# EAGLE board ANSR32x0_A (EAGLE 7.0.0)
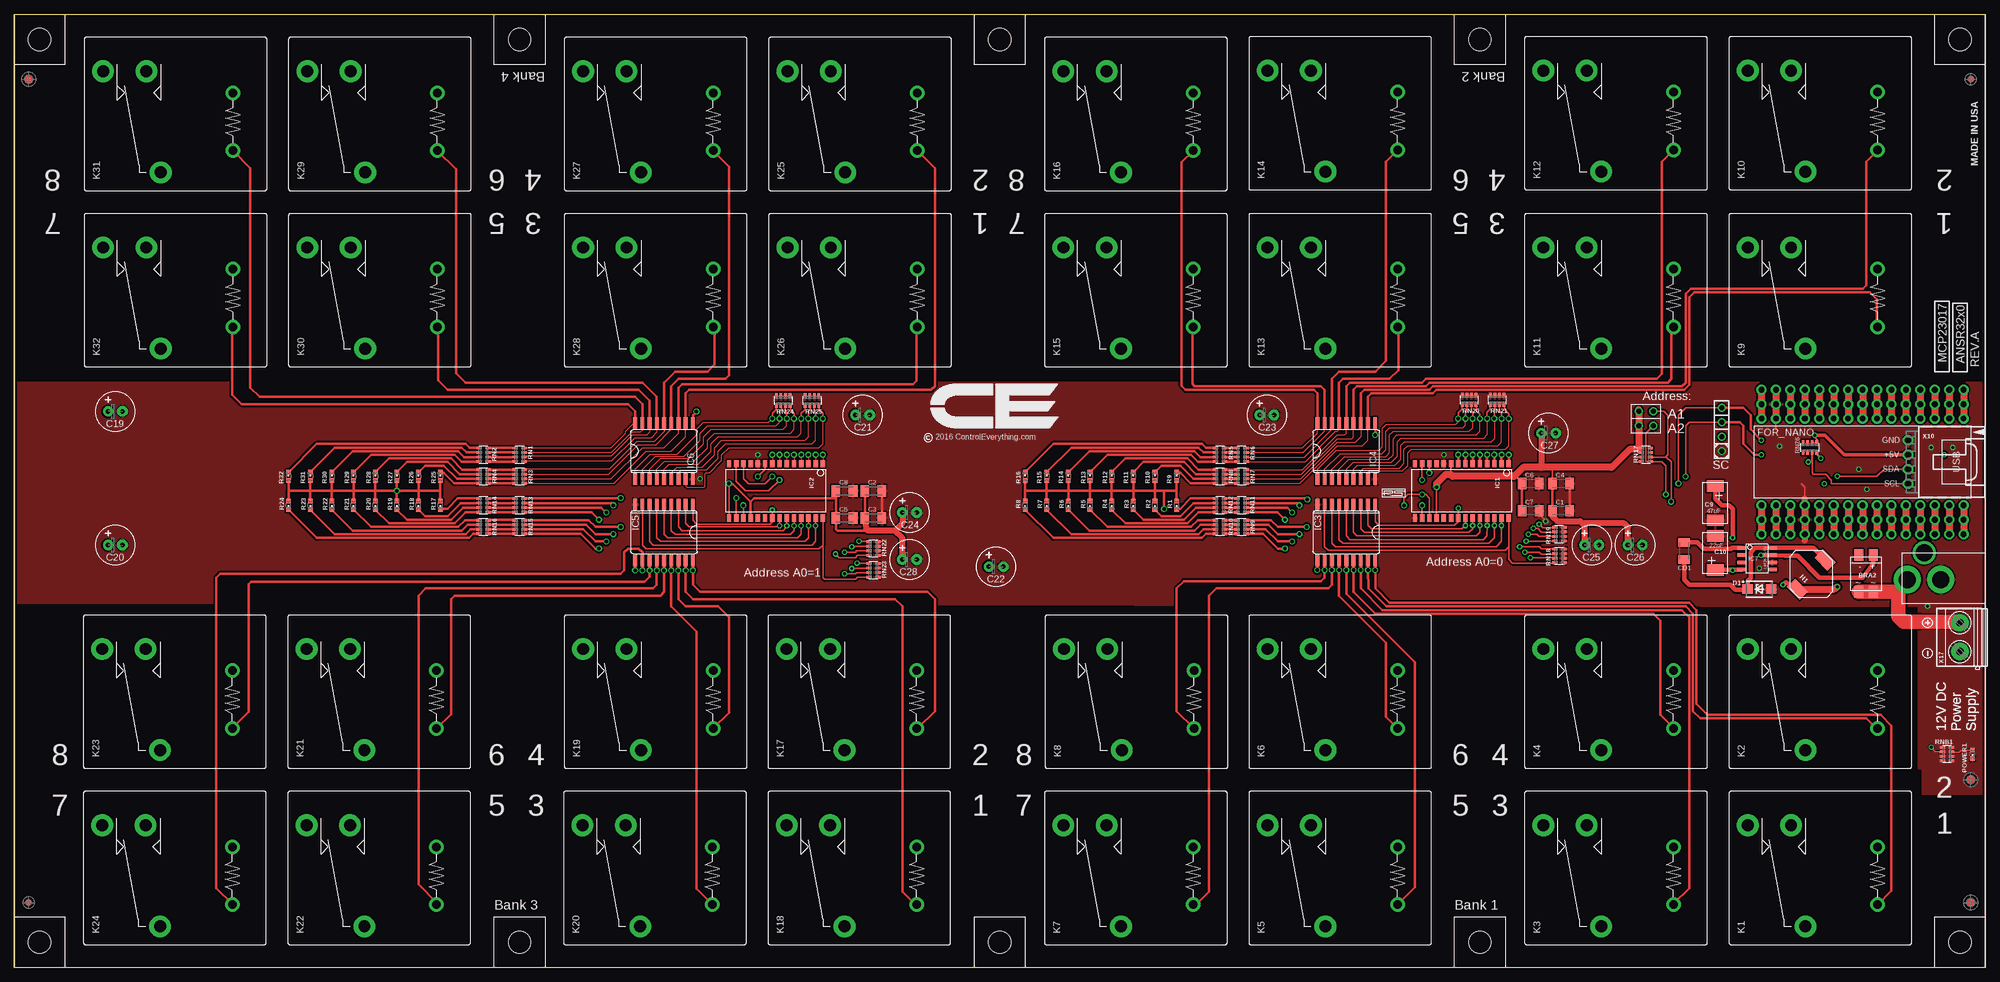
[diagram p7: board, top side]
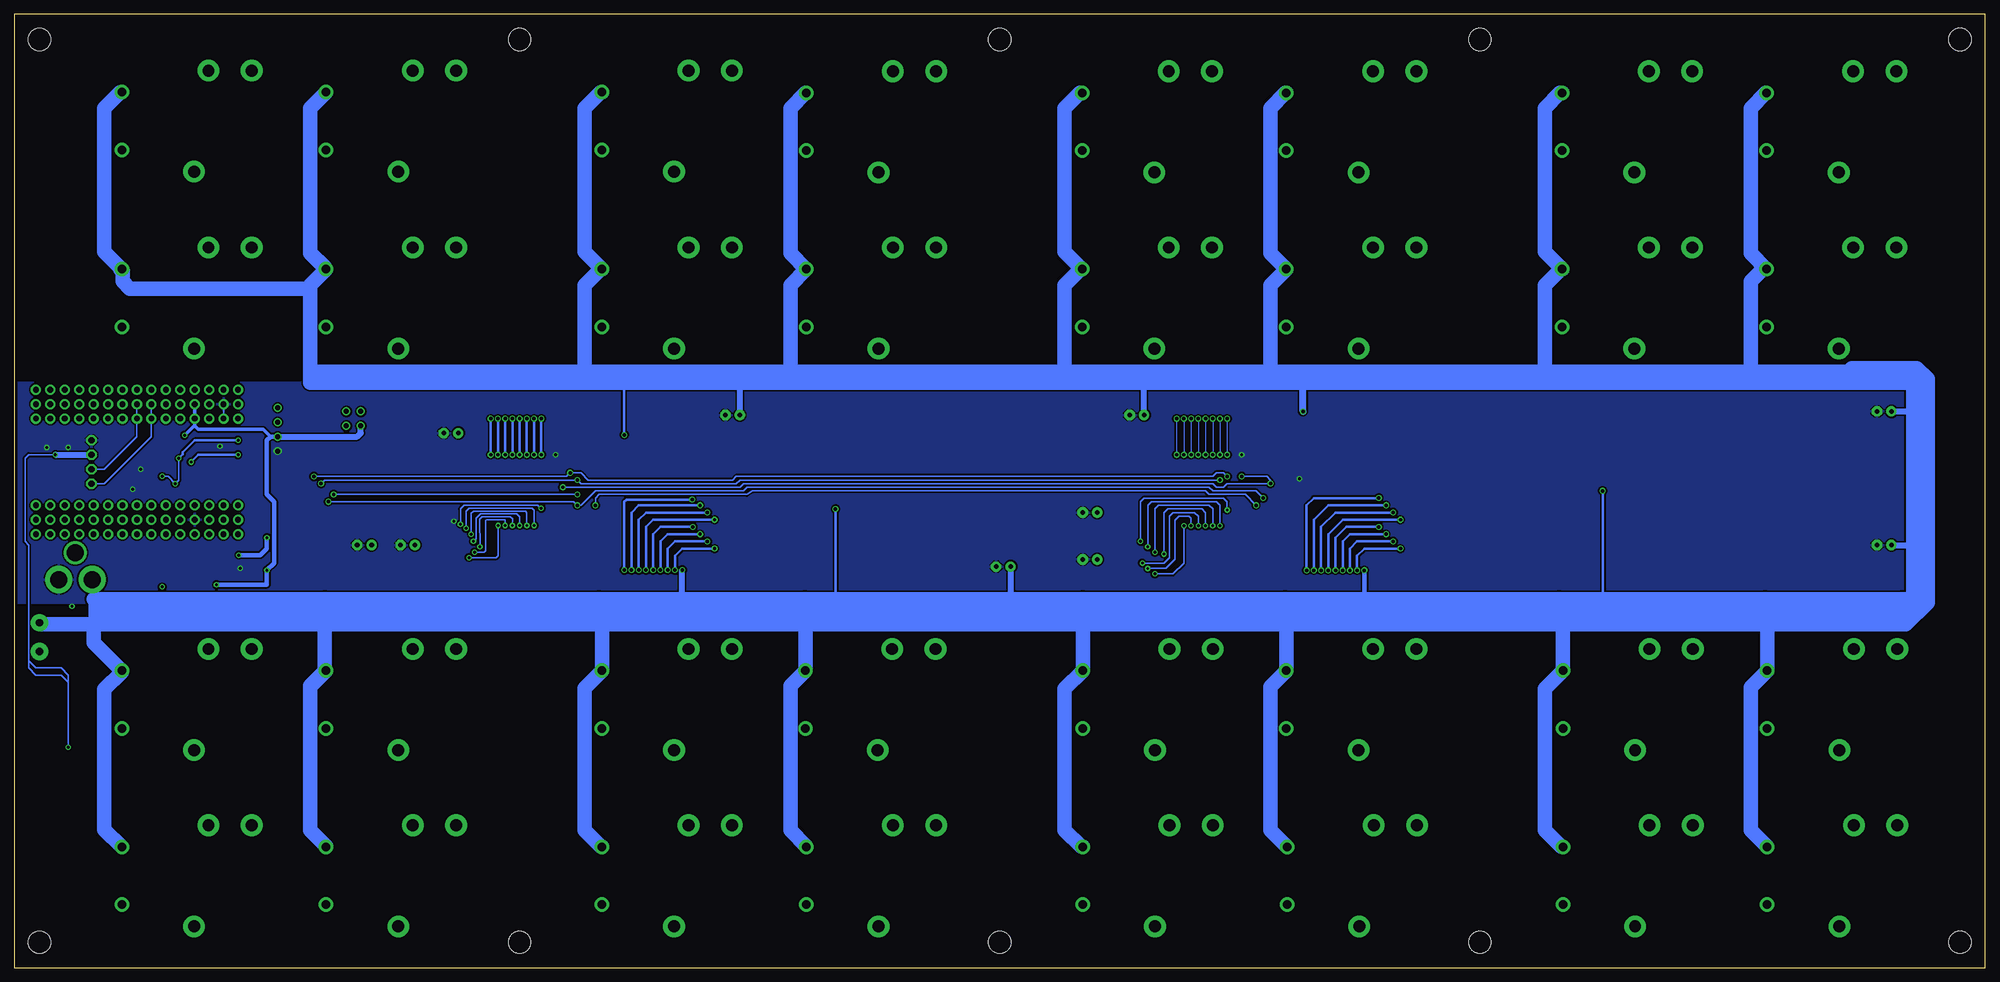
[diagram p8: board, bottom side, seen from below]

Size 346.71 x 167.65 mm. Coordinates in mm from the lower left corner, seen from the top.
Outline: 346.69,102.88 346.69,22.23
Outline: 346.71,102.88 346.71,45.1
Outline: 0,167.65 346.69,167.65 346.69,0 0,0 0,167.65
Copper layers (1*16): Top 0.035mm / dielectric 1.5mm / Bottom 0.035mm
Design rules "default *": minimum track width 6mil, minimum drill 12mil, track to track 5mil, track to pad 5mil, pad to pad 5mil, via to via 5mil, smd to smd 5mil, copper to edge 20mil, drill to drill 8mil, minimum pad ring 10mil, minimum via ring 8mil, stop-mask expansion 4mil, vias tented up to drill 0mil, thermal gap 10mil

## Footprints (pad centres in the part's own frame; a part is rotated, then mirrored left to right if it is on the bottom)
MB2S = smd 1.55 x 2.1: + 0,-6.5; - 2.54,-6.5; ~@1 0,0; ~@2 2.54,0
_CA_.1UF_50V = smd 1.5 x 2: 1 -1.5,0; 2 1.5,0
_CB_10UF_25V = smd 1.5 x 2: 1 -1.5,0; 2 1.5,0
C2917(7343)-Y = smd 2 x 3: 1 -3,0; 2 3,0
E-025X060 = drill 0.813 pad 1.778: + -1.27,0 | drill 0.813 pad 1.778 octagon: - 1.27,0
_CD_10NF_50V = smd 1.5 x 2: 1 -1.5,0; 2 1.5,0
DO214AC_ZENER = smd 1.8 x 1.7: A 2.05,0; C -2.05,0
ARDUINO_NANO = drill 1 pad 1.778: 3V1 -2.54,-2.54; 3V3 0,-2.54; 5V 0,-27.94; 5V1 -2.54,-27.94; A0 0,-7.62; A1 0,-10.16; A2 0,-12.7; A3 0,-15.24; A4 0,-17.78; A5 0,-20.32; A6 0,-22.86; A7 0,-25.4; A8 -2.54,-7.62; A9 -2.54,-10.16; A10 -2.54,-12.7; A11 -2.54,-15.24; A12 -2.54,-17.78; A13 -2.54,-20.32; A14 -2.54,-22.86; A15 -2.54,-25.4; D1 -2.54,0; D2 20.32,-25.4; D3 20.32,-22.86; D4 20.32,-20.32; D5 20.32,-17.78; D6 20.32,-15.24; D7 20.32,-12.7; D8 20.32,-10.16; D9 20.32,-7.62; D10 20.32,-5.08; D11 20.32,-2.54; D12 20.32,0; D13 0,0; D14 22.86,0; D15 22.86,-2.54; D16 22.86,-5.08; D17 22.86,-7.62; D18 22.86,-10.16; D19 22.86,-12.7; D20 22.86,-15.24; D21 22.86,-17.78; D22 22.86,-20.32; D23 22.86,-22.86; D24 22.86,-25.4; GND 0,-33.02; GND1 -2.54,-33.02; GND@1 20.32,-27.94; GND@2 22.86,-27.94; P$16 2.54,0; P$17 2.54,-2.54; P$18 2.54,-5.08; P$19 2.54,-7.62; P$20 2.54,-10.16; P$21 2.54,-12.7; P$22 2.54,-15.24; P$23 2.54,-17.78; P$24 2.54,-20.32; P$25 2.54,-22.86; P$26 2.54,-25.4; P$27 2.54,-27.94; P$28 2.54,-30.48; P$29 2.54,-33.02; P$30 2.54,-35.56; P$31 17.78,0; P$32 17.78,-2.54; P$33 17.78,-5.08; P$34 17.78,-7.62; P$35 17.78,-10.16; P$36 17.78,-12.7; P$37 17.78,-15.24; P$38 17.78,-17.78; P$39 17.78,-20.32; P$40 17.78,-22.86; P$41 17.78,-25.4; P$42 17.78,-27.94; P$43 17.78,-30.48; P$44 17.78,-33.02; P$45 17.78,-35.56; REF 0,-5.08; REF1 -2.54,-5.08; RST 0,-30.48; RST1 -2.54,-30.48; RST@1 20.32,-30.48; RST@2 22.86,-30.48; RX0 20.32,-33.02; RX1 22.86,-33.02; TX1 20.32,-35.56; TX2 22.86,-35.56; VIN 0,-35.56; VIN1 -2.54,-35.56
IND_ELL8TP = smd 2.054 x 3.2 rotated 45: 1 -2.442,-2.696; 2 2.442,2.442
SO28W = smd 0.762 x 1.27: 1 -7.62,-4.78; 2 -6.35,-4.78; 3 -5.08,-4.78; 4 -3.81,-4.78; 5 -2.54,-4.78; 6 -1.27,-4.78; 7 0,-4.78; 8 1.27,-4.78; 9 2.54,-4.78; 10 3.81,-4.78; 11 5.08,-4.78; 12 6.35,-4.78; 13 7.62,-4.78; 14 8.89,-4.78; 15 8.89,4.78; 16 7.62,4.78; 17 6.35,4.78; 18 5.08,4.78; 19 3.81,4.78; 20 2.54,4.78; 21 1.27,4.78; 22 0,4.78; 23 -1.27,4.78; 24 -2.54,4.78; 25 -3.81,4.78; 26 -5.08,4.78; 27 -6.35,4.78; 28 -7.62,4.78
SO18L = smd 0.66 x 2.032: 1 -5.08,-4.902; 2 -3.81,-4.902; 3 -2.54,-4.902; 4 -1.27,-4.902; 5 0,-4.902; 6 1.27,-4.902; 7 2.54,-4.902; 8 3.81,-4.902; 9 5.08,-4.902; 10 5.08,4.902; 11 3.81,4.902; 12 2.54,4.902; 13 1.27,4.902; 14 0,4.902; 15 -1.27,4.902; 16 -2.54,4.902; 17 -3.81,4.902; 18 -5.08,4.902
SO-8 = smd 0.6 x 1.55: 1 -1.905,-2.69; 2 -0.635,-2.69; 3 0.635,-2.69; 4 1.905,-2.69; 5 1.905,2.71; 6 0.635,2.71; 7 -0.635,2.71; 8 -1.905,2.71
JT-TMB = drill 1.5 pad 2.54: 1 5.08,0; 2 -5.08,0 | drill 2.1 pad 3.81: C -8.89,12.7; NC 8.89,22.86; NO 8.89,15.24
CHIPLED_0603 = smd 0.8 x 0.8: A 0,-0.75; C 0,0.75
RNB = smd 0.5 x 0.9: 1 -1.2,-0.8; 2 -0.4,-0.8; 3 0.4,-0.8; 4 1.2,-0.8; 5 1.2,0.8; 6 0.4,0.8; 7 -0.4,0.8; 8 -1.2,0.8
RNE = smd 0.5 x 0.9: 1 -1.2,-0.8; 2 -0.4,-0.8; 3 0.4,-0.8; 4 1.2,-0.8; 5 1.2,0.8; 6 0.4,0.8; 7 -0.4,0.8; 8 -1.2,0.8
RND = smd 0.5 x 0.9: 1 -1.2,-0.8; 2 -0.4,-0.8; 3 0.4,-0.8; 4 1.2,-0.8; 5 1.2,0.8; 6 0.4,0.8; 7 -0.4,0.8; 8 -1.2,0.8
PCB_MOUNTING_HOLE = hole 3.962: 4.445,4.445
PJ-102A = drill 3 pad 4.8: RING 0.1,-3.39; TIP 0.1,-9.29 | drill 3 pad 3.251: RING_SW -4.6,-6.29
JUMPER_2X2 = drill 0.9: A1 0,2.54; A2 0,0; B1 2.54,2.54; B2 2.54,0
70553-04 = drill 1.1 pad 1.778 octagon: 1 -3.81,-7.62; 2 -1.27,-7.62; 3 1.27,-7.62; 4 3.81,-7.62
MKDSN1,5/2-5,08 = drill 1.3 pad 3.048: 1 -2.561,0.025; 2 2.519,0.025

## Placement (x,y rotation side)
BRA2  MB2S_  [MB2S]  327.02,66.05 180 top
C1  [_CA_.1UF_50V]  272.1,80.34 0 top
C2  _CB_10UF_25VC1206K  [_CB_10UF_25V]  151.13,83.83 0 top
C3  [_CA_.1UF_50V]  151.13,79.07 0 top
C4  _CB_10UF_25VC1206K  [_CB_10UF_25V]  272.1,85.1 0 top
C5  [_CA_.1UF_50V]  146.05,79.07 0 top
C6  _CB_10UF_25VC1206K  [_CB_10UF_25V]  266.7,85.1 0 top
C7  [_CA_.1UF_50V]  266.7,80.34 0 top
C8  _CB_10UF_25VC1206K  [_CB_10UF_25V]  146.05,83.83 0 top
C9  47uF  [C2917(7343)-Y]  299.21,81.67 270 top
C10  22uF  [C2917(7343)-Y]  299.21,72.89 90 top
C19  100uF  [E-025X060]  17.78,97.8 0 top
C20  100uF  [E-025X060]  17.78,74.31 0 top
C21  100uF  [E-025X060]  149.22,97.17 0 top
C22  100uF  [E-025X060]  172.72,70.5 0 top
C23  100uF  [E-025X060]  220.34,97.17 0 top
C24  100uF  [E-025X060]  157.48,80.02 0 top
C25  100uF  [E-025X060]  277.5,74.31 0 top
C26  100uF  [E-025X060]  285.12,74.31 0 top
C27  100uF  [E-025X060]  269.88,93.99 0 top
C28  100uF  [E-025X060]  157.48,71.77 0 top
CD1  [_CD_10NF_50V]  293.75,73.29 270 top
D1  B360A  [DO214AC_ZENER]  306.96,66.56 0 top
FOR_NANO  ARDUINO_NANO  [ARDUINO_NANO]  342.9,99.07 270 top
H1  ELL8TP  [IND_ELL8TP]  316.1,69.23 0 top
IC1  MCP23017SO  [SO28W]  255.27,83.83 180 top
IC2  MCP23017SO  [SO28W]  134.62,83.83 180 top
IC3  ULN2803  [SO18L]  234.31,76.53 180 top
IC4  ULN2803  [SO18L]  234.31,90.82 0 top
IC5  ULN2803  [SO18L]  114.3,76.53 180 top
IC6  ULN2803  [SO18L]  114.3,90.82 0 top
IC7  LM2675-5V  [SO-8]  306.58,71.89 270 top
K1  JTN-TMB-DC12V  [JT-TMB]  327.79,16.14 90 top
K2  JTN-TMB-DC12V  [JT-TMB]  327.79,47.13 90 top
K3  JTN-TMB-DC12V  [JT-TMB]  291.85,16.14 90 top
K4  JTN-TMB-DC12V  [JT-TMB]  291.85,47.13 90 top
K5  JTN-TMB-DC12V  [JT-TMB]  243.33,16.14 90 top
K6  JTN-TMB-DC12V  [JT-TMB]  243.33,47.13 90 top
K7  JTN-TMB-DC12V  [JT-TMB]  207.39,16.14 90 top
K8  JTN-TMB-DC12V  [JT-TMB]  207.52,47.13 90 top
K9  JTN-TMB-DC12V  [JT-TMB]  327.79,117.74 90 top
K10  JTN-TMB-DC12V  [JT-TMB]  327.79,148.86 90 top
K11  JTN-TMB-DC12V  [JT-TMB]  291.85,117.74 90 top
K12  JTN-TMB-DC12V  [JT-TMB]  291.85,148.86 90 top
K13  JTN-TMB-DC12V  [JT-TMB]  243.33,117.74 90 top
K14  JTN-TMB-DC12V  [JT-TMB]  243.33,148.86 90 top
K15  JTN-TMB-DC12V  [JT-TMB]  207.39,117.74 90 top
K16  JTN-TMB-DC12V  [JT-TMB]  207.39,148.73 90 top
K17  JTN-TMB-DC12V  [JT-TMB]  158.75,47.13 90 top
K18  JTN-TMB-DC12V  [JT-TMB]  158.75,16.14 90 top
K19  JTN-TMB-DC12V  [JT-TMB]  122.94,47.13 90 top
K20  JTN-TMB-DC12V  [JT-TMB]  122.81,16.14 90 top
K21  JTN-TMB-DC12V  [JT-TMB]  74.3,47.13 90 top
K22  JTN-TMB-DC12V  [JT-TMB]  74.3,16.14 90 top
K23  JTN-TMB-DC12V  [JT-TMB]  38.35,47.13 90 top
K24  JTN-TMB-DC12V  [JT-TMB]  38.35,16.14 90 top
K25  JTN-TMB-DC12V  [JT-TMB]  158.88,148.73 90 top
K26  JTN-TMB-DC12V  [JT-TMB]  158.88,117.74 90 top
K27  JTN-TMB-DC12V  [JT-TMB]  122.94,148.73 90 top
K28  JTN-TMB-DC12V  [JT-TMB]  122.94,117.74 90 top
K29  JTN-TMB-DC12V  [JT-TMB]  74.42,148.73 90 top
K30  JTN-TMB-DC12V  [JT-TMB]  74.42,117.74 90 top
K31  JTN-TMB-DC12V  [JT-TMB]  38.48,148.73 90 top
K32  JTN-TMB-DC12V  [JT-TMB]  38.48,117.74 90 top
POWER1  LED_NCD  [CHIPLED_0603]  344.49,37.48 180 top
R1  LED_NCD  [CHIPLED_0603]  204.47,81.29 180 top
R2  LED_NCD  [CHIPLED_0603]  200.66,81.29 180 top
R3  LED_NCD  [CHIPLED_0603]  196.85,81.29 180 top
R4  LED_NCD  [CHIPLED_0603]  193.04,81.29 180 top
R5  LED_NCD  [CHIPLED_0603]  189.23,81.29 180 top
R6  LED_NCD  [CHIPLED_0603]  185.42,81.29 180 top
R7  LED_NCD  [CHIPLED_0603]  181.61,81.29 180 top
R8  LED_NCD  [CHIPLED_0603]  177.8,81.29 180 top
R9  LED_NCD  [CHIPLED_0603]  204.47,86.37 0 top
R10  LED_NCD  [CHIPLED_0603]  200.66,86.37 0 top
R11  LED_NCD  [CHIPLED_0603]  196.85,86.37 0 top
R12  LED_NCD  [CHIPLED_0603]  193.04,86.37 0 top
R13  LED_NCD  [CHIPLED_0603]  189.23,86.37 0 top
R14  LED_NCD  [CHIPLED_0603]  185.42,86.37 0 top
R15  LED_NCD  [CHIPLED_0603]  181.61,86.37 0 top
R16  LED_NCD  [CHIPLED_0603]  177.8,86.37 0 top
R17  LED_NCD  [CHIPLED_0603]  74.93,81.29 180 top
R18  LED_NCD  [CHIPLED_0603]  71.12,81.29 180 top
R19  LED_NCD  [CHIPLED_0603]  67.31,81.29 180 top
R20  LED_NCD  [CHIPLED_0603]  63.5,81.29 180 top
R21  LED_NCD  [CHIPLED_0603]  59.69,81.29 180 top
R22  LED_NCD  [CHIPLED_0603]  55.88,81.29 180 top
R23  LED_NCD  [CHIPLED_0603]  52.07,81.29 180 top
R24  LED_NCD  [CHIPLED_0603]  48.26,81.29 180 top
R25  LED_NCD  [CHIPLED_0603]  74.93,86.37 0 top
R26  LED_NCD  [CHIPLED_0603]  71.12,86.37 0 top
R27  LED_NCD  [CHIPLED_0603]  67.31,86.37 0 top
R28  LED_NCD  [CHIPLED_0603]  63.5,86.37 0 top
R29  LED_NCD  [CHIPLED_0603]  59.69,86.37 0 top
R30  LED_NCD  [CHIPLED_0603]  55.88,86.37 0 top
R31  LED_NCD  [CHIPLED_0603]  52.07,86.37 0 top
R32  LED_NCD  [CHIPLED_0603]  48.26,86.37 0 top
RN1  _RNB_510  [RNB]  88.9,90.18 90 top
RN2  _RNB_510  [RNB]  82.55,90.18 90 top
RN3  _RNB_510  [RNB]  88.9,86.37 270 top
RN4  _RNB_510  [RNB]  82.55,86.37 270 top
RN5  _RNB_510  [RNB]  212.09,90.18 270 top
RN6  _RNB_510  [RNB]  215.9,90.18 270 top
RN7  _RNB_510  [RNB]  215.9,86.37 270 top
RN8  _RNB_510  [RNB]  212.09,86.37 270 top
RN9  _RNB_510  [RNB]  215.9,77.48 270 top
RN10  _RNB_510  [RNB]  212.09,77.48 270 top
RN11  _RNB_510  [RNB]  215.9,81.29 90 top
RN12  _RNB_510  [RNB]  212.09,81.29 90 top
RN13  _RNB_510  [RNB]  88.9,81.29 270 top
RN14  _RNB_510  [RNB]  82.55,81.29 270 top
RN15  _RNB_510  [RNB]  88.9,77.48 270 top
RN16  _RNB_510  [RNB]  82.55,77.48 270 top
RN17  _RNE_10K  [RNE]  287.02,90.18 270 top
RN18  _RNE_10K  [RNE]  271.78,72.4 90 top
RN19  _RNE_10K  [RNE]  271.78,76.21 90 top
RN20  _RNE_10K  [RNE]  255.91,99.83 180 top
RN21  _RNE_10K  [RNE]  260.86,99.83 180 top
RN22  _RNE_10K  [RNE]  151.13,73.67 90 top
RN23  _RNE_10K  [RNE]  151.13,69.86 90 top
RN24  _RNE_10K  [RNE]  135.25,99.71 180 top
RN25  _RNE_10K  [RNE]  140.34,99.71 180 top
RN26  _RND_4.7K  [RND]  315.85,91.45 0 top
RNB1  _RNB_510  [RNB]  339.98,37.54 90 top
U$1  PCB_MOUNTING_HOLE  [PCB_MOUNTING_HOLE]  262.25,158.76 90 top
U$2  2.1MMJACK  [PJ-102A]  342.26,68.34 270 top
U$3  PCB_MOUNTING_HOLE  [PCB_MOUNTING_HOLE]  346.71,158.76 90 top
U$4  PCB_MOUNTING_HOLE  [PCB_MOUNTING_HOLE]  84.45,8.9 270 top
U$5  PCB_MOUNTING_HOLE  [PCB_MOUNTING_HOLE]  168.91,8.9 270 top
U$6  PCB_MOUNTING_HOLE  [PCB_MOUNTING_HOLE]  0,8.9 270 top
U$7  PCB_MOUNTING_HOLE  [PCB_MOUNTING_HOLE]  93.34,158.76 90 top
U$8  PCB_MOUNTING_HOLE  [PCB_MOUNTING_HOLE]  8.89,158.76 90 top
U$9  PCB_MOUNTING_HOLE  [PCB_MOUNTING_HOLE]  177.8,158.76 90 top
U$10  PCB_MOUNTING_HOLE  [PCB_MOUNTING_HOLE]  253.37,8.9 270 top
U$11  PCB_MOUNTING_HOLE  [PCB_MOUNTING_HOLE]  337.82,8.9 270 top
U$12  PCB_MOUNTING_HOLE  [PCB_MOUNTING_HOLE]  168.91,8.9 270 top
U$13  JUMPER_2X2  [JUMPER_2X2]  285.75,97.8 270 top
U$15  [VISION_REF15]  344.17,11.44 90 top
U$17  [ICON_MINUS]  336.55,55.26 90 top
U$18  [VISION_REF10]  344.17,156.22 90 top
U$19  [ICON_PLUS]  336.55,60.66 0 top
U$20  [VISION_REF15]  344.17,33.03 90 top
U$21  [ICON_USA]  345.44,140.98 90 top
U$22  [ICON_MINUS]  336.55,55.26 90 top
U$23  [VISION_REF15]  2.54,156.22 90 top
U$24  [ICON_PLUS]  336.55,60.66 0 top
U$25  [ICON_MINUS]  336.55,55.26 90 top
U$26  [ICON_PLUS]  336.55,60.66 0 top
U$28  [VISION_REF10]  2.54,11.44 90 top
X10  C-GRID-04-70553  [70553-04]  340.74,88.91 270 top
X17  MKDSN1,5/2-5,08  [MKDSN1,5/2-5,08]  342.26,58.12 90 top

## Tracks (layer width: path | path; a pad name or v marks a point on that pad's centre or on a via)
GND  (via drill 0.5, 0.9)
  Top 0.254: 314.96,82.44 314.96,84.47 314.32,85.1 | FOR_NANO.GND@1 314.96,77.48 | 309.88,101.61 309.88,94.63
  Top 0.406: C1.2 C4.2 | C3.2 C2.2 | v269.37,78.5 269.37,78.63 268.61,79.39 268.61,79.94 C7.2
  Top 1.016: X10.1 332.97,92.72 | 314.96,75.07 314.96,81.29 314.96,82.44
  Bottom 0.254: 309.88,96.53 FOR_NANO.GND
  other vias: 336.55,63.51 120.65,85.99 251.46,90.18 130.81,90.18 300.36,90.82 337.19,91.45 310.51,91.71 341,91.45 324.49,87.64 325.88,84.09 306.96,70.24
  pour Top (isolate 0.305): -1.91,64.15 -1.91,102.88 346.39,102.88 346.39,63.51
  pour Top (isolate 0.305): 346.39,51.45 334.96,51.45 334.96,63.51 346.39,63.51
  pour Bottom (isolate 0.305): -3.17,102.88 346.07,102.88 346.07,64.15 -3.17,64.15
  pour Top (isolate 0.305): 346.39,34.94 334.96,34.94 334.96,63.51 346.39,63.51
  pour Top: 346.39,30.49 335.6,30.49 335.6,63.51 346.39,63.51
I2C_SCL  (via drill 0.5, 0.6, 0.9)
  Top 0.254: v300.36,95.9 294.64,95.9 294,95.26 v294,86.37 | X10.4 319.66,85.1 319.66,85.74 318.64,86.75 316.48,86.75 316.25,86.99 RN26.3 316.23,90.63 316.23,88.91 v315.6,88.91
  Top 0.305: IC2.12 128.27,86 129.17,85.1 132.08,85.1 v133.35,86.37 | v248.92,87.01 IC1.12
  Top 0.406: v300.36,95.9 303.53,95.9 304.17,95.26 304.17,92.09 306.07,90.18 v307.34,90.18
  Bottom 0.254: 322.58,96.53 FOR_NANO.A5
  Bottom 0.305: v294,86.37 249.56,86.37 v248.92,87.01 247.01,87.01 245.75,85.74 220.34,85.74 219.71,86.37 135.89,86.37 135.25,87.01 133.99,87.01 v133.35,86.37 | 322.58,96.53 322.58,93.36 330.83,85.1 X10.4
  Bottom 0.406: v307.34,90.18 314.32,90.18 v315.6,88.91
I2C_SDA  (via drill 0.5, 0.6, 0.9)
  Top 0.254: v300.36,98.44 294,98.44 292.74,97.17 v292.74,85.1 | RN26.4 317.05,90.25 v317.75,89.55 | v318.38,85.09 v318.39,85.1 | X10.3 328.93,87.64 327.66,86.37 v320.68,86.37
  Top 0.305: IC2.13 127,85.49 128.66,83.83 132.72,83.83 v134.62,85.74 | v247.65,85.74 IC1.13
  Top 0.406: v300.36,98.44 304.17,98.44 305.44,97.17 305.44,94.63 v307.34,92.72
  Bottom 0.254: v317.75,89.55 317.75,85.74 v318.39,85.1 319.66,86.37 v320.68,86.37
  Bottom 0.305: v134.62,85.74 219.07,85.74 219.71,85.1 247.01,85.1 v247.65,85.74 292.1,85.74 v292.74,85.1 | FOR_NANO.A4 325.12,93.36 330.83,87.64 X10.3
  Bottom 0.406: v307.34,92.72 314.98,92.72 RN26.4 317.05,90.25 v317.75,89.55
N$10  (via drill 0.6)
  Top 0.305: 204.47,83.83 R1.A
  Top 0.406: IC5.10 v109.22,69.86 | IC6.10 119.38,97.17 v120.02,97.8 | IC4.10 v239.4,93.68 | R8.A 177.8,83.83 | R15.A 181.61,83.83 | R6.A 185.42,83.83 | 189.23,83.83 R13.A | R4.A 193.04,83.83 | R3.A 196.85,83.83 | R2.A 200.66,83.83 | R16.A 177.8,83.83 | 177.8,83.83 181.61,83.83 | R7.A 181.61,83.83 | 181.61,83.83 185.42,83.83 | R14.A 185.42,83.83 | 185.42,83.83 189.23,83.83 | R5.A 189.23,83.83 | 189.23,83.83 193.04,83.83 | R12.A 193.04,83.83 | 193.04,83.83 196.85,83.83 | R11.A 196.85,83.83 | 196.85,83.83 200.66,83.83 | R10.A 200.66,83.83 | R24.A 48.26,83.83 | R31.A 52.07,83.83 | R30.A 55.88,83.83 | R29.A 59.69,83.83 | R28.A 63.5,83.83 | v67.31,83.83 R19.A | 71.12,83.83 R18.A | R25.A 74.93,83.83 | 74.93,83.83 R17.A | R32.A 48.26,83.83 | 48.26,83.83 52.07,83.83 | R23.A 52.07,83.83 | 52.07,83.83 55.88,83.83 | R22.A 55.88,83.83 | 55.88,83.83 59.69,83.83 | R21.A 59.69,83.83 | 59.69,83.83 63.5,83.83 | R20.A 63.5,83.83 | 63.5,83.83 v67.31,83.83 | v67.31,83.83 71.12,83.83 | R26.A 71.12,83.83 | 71.12,83.83 74.93,83.83 | R9.A 204.47,83.83 | 204.47,81.93 204.47,83.83 | 204.47,83.83 202.25,83.83 | 200.66,83.83 202.25,83.83 | 202.25,83.83 v202.25,80.66 | IC3.10 229.24,70.5 v229.2,69.93 | R27.A v67.31,83.83
  Bottom 0.305: 327.66,122.57 327.66,122.69 K9.1
  Bottom 0.406: v239.4,93.68 239.4,102.25 238.76,102.88 | v202.25,80.66 202.25,64.78 | 229.3,65.1 229.62,64.78 | v67.31,83.83 67.31,64.78
  Bottom 0.813: v109.22,69.86 109.22,64.78
  Bottom 1.016: 229.3,65.1 229.2,65.1 v229.2,69.93 | 220.34,102.25 219.71,102.88 | 31.11,102.25 31.75,102.88 | C22.+ 171.45,65.42 170.81,64.78 | C23.+ 219.07,102.88 | C21.+ 147.96,102.88 | C20.+ 12.7,74.31 | C19.+ 12.7,97.8
  Bottom 1.27: v120.02,97.8 120.02,102.88
  Bottom 2.54: 327.66,122.57 327.66,120.66 326.39,119.39 294.64,119.39 | 332.74,64.78 332.36,64.4 332.36,60.97 332.7,60.63 332.7,57.12 K2.1 327.79,51.96 330.83,48.91 330.83,24.27 K1.1 | 332.74,64.78 292.1,64.78 | 292.1,64.78 243.84,64.78 | 243.84,64.78 229.62,64.78 207.65,64.78 | 207.65,64.78 202.25,64.78 170.81,64.78 158.75,64.78 | 158.75,64.78 123.19,64.78 | 123.19,64.78 109.22,64.78 74.93,64.78 | 74.93,64.78 67.31,64.78 38.73,64.78 | 38.73,64.78 14.61,64.78 | 41.27,102.88 31.75,102.88 12.7,102.88 12.7,97.8 12.7,74.31 12.7,64.78 | 41.27,102.88 77.47,102.88 | 77.47,102.88 120.02,102.88 126.36,102.88 | 126.36,102.88 147.96,102.88 161.93,102.88 | 161.93,102.88 210.19,102.88 | 210.19,102.88 219.07,102.88 219.71,102.88 238.76,102.88 246.38,102.88 | 246.38,102.88 294.64,102.88 294.64,104.79 | 332.13,64.44 332.74,64.78 | K3.1 291.85,21.35 294.64,24.14 294.64,49.42 | 294.64,49.42 K4.1 | K5.1 243.46,21.22 246.38,24.14 246.38,49.16 K6.1 243.33,64.27 243.84,64.78 | K7.1 207.39,21.35 210.19,24.14 210.19,49.54 K8.1 207.52,64.66 207.65,64.78 | K18.1 159,21.22 161.93,24.14 161.93,49.03 K17.1 158.75,64.78 | K20.1 125.73,24.14 125.73,49.42 K19.1 122.94,64.53 123.19,64.78 | K22.1 74.55,21.22 77.47,24.14 77.47,49.03 K21.1 74.3,64.15 74.93,64.78 | K24.1 41.27,24.14 41.27,49.29 K23.1 38.35,64.4 38.73,64.78 | 294.64,49.42 294.64,49.54 292.1,52.08 292.1,64.78 | K12.1 294.64,151.14 294.64,125.74 | 294.64,125.74 294.64,125.62 K11.1 | K10.1 328.04,153.94 330.83,151.14 330.83,125.87 K9.1 328.04,122.82 | K14.1 243.59,153.94 246.38,151.14 246.38,125.87 K13.1 243.59,122.82 246.38,120.03 246.38,102.88 | K16.1 207.52,153.81 210.19,151.14 210.19,125.62 K15.1 210.19,120.03 210.19,102.88
  Bottom 2.54: K25.1 159.26,153.81 161.93,151.14 161.93,125.87 K26.1 159.13,122.82 161.93,120.03 161.93,102.88 | K27.1 123.06,153.81 125.73,151.14 125.73,125.62 K28.1 125.73,120.03 125.73,103.52 126.36,102.88 | K29.1 74.8,153.81 77.47,151.14 77.47,125.87 K30.1 74.68,122.82 77.47,120.03 77.47,102.88 | K31.1 38.61,153.81 41.27,151.14 41.27,125.62 K32.1 39.12,122.82 41.27,120.66 41.27,102.88 | 294.64,125.74 292.1,123.2 292.1,122.57 294.64,120.03 294.64,119.39 | 294.64,119.39 294.64,104.79 | 17.14,60.34 331.47,60.34 342.26,60.34 | 17.14,60.34 12.7,64.78 | 12.7,64.78 14.61,64.78 | 14.61,64.78 17.14,62.24 330.83,62.24 330.83,63.51 20.32,63.51 17.14,60.34 | 17.14,60.34 13.97,60.34 10.16,64.15 10.16,103.52 12.06,105.42 23.5,105.42 24.13,104.79 294.64,104.79
N$99
  Top 0.254: POWER1.A 342.51,38.23 342.14,37.86 340.86,37.86 RNB1.3
  Top 0.406: 340.82,37.99 RNB1.3
N$100
  Top 0.813: 307.98,73.8 IC7.8 316.42,73.8 H1.2 | 307.98,73.8 306.2,73.8 305.44,73.04 305.44,68.49 304.93,67.98 304.93,66.58 D1.C 304.78,66.43 302.77,66.43 301.88,67.32 294.64,67.32 293.75,68.21 CD1.2 | 307.95,73.82 307.98,73.8
N$101
  Top 0.813: CD1.1 296.06,74.79 297.18,73.67 302.01,73.67 302.13,73.8 IC7.1
N$405  (via drill 0.5)
  Top 0.229: IC1.21 254,78.44 253.37,77.8 240.03,77.8 239.4,78.44 IC3.1
  Top 0.254: 254,78.44 v254,80.78 | v268.22,77.99 268.86,77.36 270.92,77.36
  Top 0.305: 270.92,77.36 270.98,77.36 RN19.5
  Bottom 0.229: v254,80.78 254,80.66 254.63,81.29 267.59,81.29 268.22,80.66 v268.22,77.99
N$406  (via drill 0.5)
  Top 0.229: IC1.25 v259.09,77.74 259.08,75.89 258.44,75.26 234.95,75.26 234.31,75.89 IC3.5 | v264.8,73.99 268.29,73.99 268.61,73.67 270.91,73.67 RN18.5
  Bottom 0.229: v259.09,77.74 259.08,78.9 259.44,79.26 264.39,79.26 264.8,78.86 v264.8,73.99
N$407  (via drill 0.5)
  Top 0.229: IC1.26 v260.35,77.74 260.35,75.58 259.4,74.63 233.68,74.63 233.04,75.26 IC3.6 | v265.75,73.04 268.29,73.04 268.61,72.72 270.9,72.72 RN18.6
  Bottom 0.229: v260.35,77.74 260.35,78.63 260.48,78.75 263.65,78.75 263.78,78.63 263.78,73.29 264.03,73.04 v265.75,73.04
N$408  (via drill 0.6)
  Top 0.305: IC2.16 v127,82.56 | v247.65,81.29 IC1.16 | RN17.6 290.43,89.78 | 290.43,89.78 290.83,90.18 290.83,97.17 290.19,97.8 U$13.A1 | 290.43,89.78 290.6,89.78 291.46,88.91 v291.46,81.93
  Bottom 0.305: v127,82.56 128.27,83.83 135.89,83.83 136.53,84.47 217.81,84.47 218.44,83.83 244.47,83.83 247.01,81.29 v247.65,81.29 248.28,81.93 v291.46,81.93
N$409  (via drill 0.5)
  Top 0.229: IC1.22 255.27,77.8 254.63,77.16 238.76,77.16 238.12,77.8 IC3.2
  Top 0.254: 255.27,77.8 v255.27,77.74 | v267.21,77.23 267.97,77.23 268.61,76.59 270.96,76.59 RN19.6
  Bottom 0.229: v255.27,77.74 255.27,80.4 255.65,80.78 266.7,80.78 267.21,80.28 v267.21,77.23
N$410  (via drill 0.5)
  Top 0.229: IC1.23 256.54,77.16 255.91,76.53 237.49,76.53 236.85,77.16 IC3.3
  Top 0.254: 256.54,77.16 v256.54,77.74 | v266.32,76.21 267.84,76.21 268.22,75.83 270.96,75.83 RN19.7
  Bottom 0.229: v256.54,77.74 256.54,80.02 256.79,80.28 265.94,80.28 266.32,79.9 v266.32,76.21
  Bottom 0.254: 266.57,76.09 v266.32,76.21
N$411  (via drill 0.5)
  Top 0.229: IC1.24 257.81,76.53 257.18,75.89 236.22,75.89 235.59,76.53 IC3.4
  Top 0.254: 257.81,76.53 v257.81,77.74 | v265.94,74.94 270.91,74.94 RN19.8
  Bottom 0.229: v257.81,77.74 257.81,79.26 258.32,79.77 264.67,79.77 265.43,79.01 265.43,75.45 v265.94,74.94
N$416  (via drill 0.6)
  Top 0.203: 238.12,87.01 238.44,87.32 244.16,87.32 245.11,88.28 245.11,90.5 245.75,91.13 262.25,91.13 262.89,91.77 v262.89,96.53
  Top 0.229: v262.89,96.53 262.89,97.42 262.13,98.18 262.13,98.96 RN21.8
  Top 0.406: v262.89,90.18 IC1.1 | IC4.8 238.12,87.01
  Bottom 0.406: v262.89,96.53 v262.89,90.18
N$417  (via drill 0.6)
  Top 0.203: IC4.7 236.85,87.32 237.36,87.83 243.65,87.83 244.47,88.66 244.47,91.13 245.11,91.77 260.99,91.77 261.62,92.4 v261.62,96.53
  Top 0.229: v261.62,96.53 261.62,97.55 261.24,97.93 261.24,99.02 RN21.7
  Top 0.406: v261.62,90.18 IC1.2
  Bottom 0.406: v261.62,96.53 v261.62,90.18
N$418  (via drill 0.6)
  Top 0.203: IC4.6 235.59,87.64 236.28,88.34 242.89,88.34 243.84,89.29 243.84,91.77 244.47,92.4 259.71,92.4 260.35,93.04 v260.35,96.53
  Top 0.229: v260.35,96.53 260.35,98.06 260.48,98.18 260.48,99.02 RN21.6
  Top 0.406: v260.35,90.18 IC1.3
  Bottom 0.406: v260.35,96.53 v260.35,90.18
N$419  (via drill 0.6)
  Top 0.203: IC4.5 234.31,87.64 235.52,88.85 242.25,88.85 243.21,89.8 243.21,92.4 243.84,93.04 258.44,93.04 259.08,93.68 v259.08,96.53
  Top 0.229: v259.08,96.53 259.08,97.68 259.59,98.18 259.59,98.96 RN21.5
  Top 0.406: v259.08,90.18 IC1.4
  Bottom 0.406: v259.08,90.18 v259.08,96.53
N$420  (via drill 0.6)
  Top 0.203: IC4.4 233.04,87.64 234.76,89.36 241.74,89.36 242.57,90.18 242.57,93.04 243.21,93.68 257.18,93.68 257.81,94.31 v257.81,96.53
  Top 0.229: v257.81,96.53 257.81,97.29 257.18,97.93 257.18,98.96 RN20.8
  Top 0.406: v257.81,90.18 IC1.5
  Bottom 0.406: v257.81,96.53 v257.81,90.18
N$421  (via drill 0.6)
  Top 0.203: IC4.3 231.78,87.64 234,89.87 241.24,89.87 241.94,90.56 241.94,93.68 242.57,94.31 255.91,94.31 256.54,94.95 v256.54,96.53
  Top 0.229: v256.54,96.53 256.54,97.68 256.29,97.93 256.29,99.02 RN20.7
  Top 0.406: v256.54,90.18 IC1.6
  Bottom 0.406: v256.54,96.53 v256.54,90.18
N$422  (via drill 0.6)
  Top 0.203: IC4.2 230.5,87.64 233.24,90.37 240.6,90.37 241.3,91.07 241.3,94.31 241.94,94.95 254.82,94.95 255.27,95.39 v255.27,96.53
  Top 0.229: IC1.7 255.27,88.28 | v255.27,96.53 255.27,97.55 255.52,97.8 255.52,99.02 RN20.6
  Top 0.406: 255.27,96.16 v255.27,96.53 | v255.27,90.18 IC1.7
  Bottom 0.406: v255.27,96.53 v255.27,90.18
N$423  (via drill 0.6)
  Top 0.203: IC4.1 229.24,87.64 232.6,91.01 240.09,91.01 240.66,91.58 240.66,94.87 241.38,95.58 253.55,95.58 254,96.03 v254,96.53
  Top 0.229: v254,96.53 254,97.55 254.63,98.18 254.63,98.96 RN20.5
  Top 0.406: v254,90.18 IC1.8
  Bottom 0.406: v254,90.18 v254,96.53
N$424  (via drill 0.5)
  Top 0.229: IC2.21 v133.35,80.47 133.35,78.38 132.96,77.99 120.02,77.99 119.38,78.63 IC5.1 | v148.59,74.94 150.26,74.94 RN22.5
  Bottom 0.229: v133.35,80.47 133.35,81.93 133.99,82.56 147.96,82.56 148.59,81.93 v148.59,74.94
N$425  (via drill 0.5)
  Top 0.229: IC5.2 118.11,78.12 118.75,77.48 134.62,77.48 v134.62,77.67 IC2.22 | RN22.6 147.4,74.07 v147.32,73.99
  Bottom 0.229: v147.32,73.99 147.32,81.29 146.69,81.93 135.25,81.93 134.62,81.29 v134.62,77.67
N$426  (via drill 0.5)
  Top 0.229: IC5.3 116.84,77.48 117.47,76.85 135.25,76.85 135.89,77.48 v135.89,77.67 IC2.23 | RN22.7 148.19,73.27 147.96,73.04 v146.05,73.04
  Bottom 0.229: v146.05,73.04 146.05,80.66 145.41,81.29 136.53,81.29 135.89,80.66 v135.89,77.67
N$427  (via drill 0.5)
  Top 0.229: IC5.4 115.57,76.85 116.2,76.21 136.53,76.21 137.16,76.85 v137.16,77.67 IC2.24 | RN22.8 148.34,72.47 147.96,72.09 145.1,72.09 v144.46,72.72
  Bottom 0.229: v144.46,72.72 144.46,79.95 143.75,80.66 137.79,80.66 137.16,80.02 v137.16,77.67
N$428  (via drill 0.5)
  Top 0.229: IC5.5 114.3,76.21 114.94,75.58 137.79,75.58 138.43,76.21 v138.43,77.67 IC2.25 | RN23.5 148.34,71.06 v148.27,71.13
  Bottom 0.229: v148.27,71.13 144.46,71.13 143.51,72.09 143.51,79.39 142.88,80.02 139.06,80.02 138.43,79.39 v138.43,77.67
N$429  (via drill 0.5)
  Top 0.229: IC5.6 113.03,75.58 113.67,74.94 139.06,74.94 139.7,75.58 v139.7,77.67 IC2.26 | RN23.6 147.4,70.26 v147.32,70.18
  Bottom 0.229: v147.32,70.18 144.15,70.18 142.56,71.77 142.56,78.68 141.85,79.39 140.03,79.39 IC2.26 v139.7,77.67
N$430  (via drill 0.5)
  Top 0.229: IC5.7 111.76,74.94 112.39,74.31 140.34,74.31 140.97,74.94 v140.97,77.67 IC2.27 | RN23.7 148.19,69.46 147.96,69.23 v146.05,69.23
  Bottom 0.229: v146.05,69.23 142.88,69.23 140.97,71.13 v140.97,77.67
N$431
  Top 0.229: IC2.28 142.24,74.31 | 142.24,74.31 141.6,73.67 111.12,73.67 110.49,74.31 IC5.8 | RN23.8 148.34,68.66 147.96,68.27 142.56,68.27 142.24,68.59 142.24,74.31
N$432  (via drill 0.6)
  Top 0.203: IC6.8 118.11,84.75 118.39,84.47 121.36,84.47 121.54,84.65 121.54,86.83 121.72,87.01 122.27,87.01 124.46,89.2 124.46,90.18 125.73,91.45 141.6,91.45 142.24,92.09 v142.24,96.53 | v142.24,90.18 IC2.1
  Top 0.229: v142.24,96.53 142.24,97.48 141.6,98.12 141.6,98.84 RN25.8
  Bottom 0.203: v142.24,96.53 v142.24,90.18
N$433  (via drill 0.6)
  Top 0.203: IC6.7 116.84,87.01 117.35,87.52 121.79,87.52 123.83,89.55 123.83,90.82 125.09,92.09 140.34,92.09 140.97,92.72 v140.97,96.53 | v140.97,90.18 IC2.2
  Top 0.229: v140.97,96.53 140.97,97.8 140.65,98.12 140.65,98.82 RN25.7
  Bottom 0.203: v140.97,96.53 v140.97,90.18
N$434  (via drill 0.6)
  Top 0.203: IC6.6 115.57,87.01 116.59,88.02 121.03,88.02 123.19,90.18 123.19,91.45 124.46,92.72 139.06,92.72 139.7,93.36 v139.7,96.53 | v139.7,90.18 IC2.3
  Top 0.229: v139.7,96.53 139.7,97.8 140.02,98.12 140.02,98.82 RN25.6
  Bottom 0.203: v139.7,96.53 v139.7,90.18
N$435  (via drill 0.6)
  Top 0.203: IC6.5 114.3,87.64 115.19,88.53 120.27,88.53 122.56,90.82 122.56,92.09 123.83,93.36 137.79,93.36 138.43,93.99 v138.43,96.53 | v138.43,90.18 IC2.4
  Top 0.229: v138.43,96.53 138.43,97.48 139.06,98.12 139.06,98.84 RN25.5
  Bottom 0.203: v138.43,96.53 v138.43,90.18
N$436  (via drill 0.6)
  Top 0.203: IC6.4 113.03,87.64 114.43,89.04 119.51,89.04 121.92,91.45 121.92,92.72 123.19,93.99 136.53,93.99 137.16,94.63 v137.16,96.53 | v137.16,90.18 IC2.5
  Top 0.229: v137.16,96.53 137.16,97.48 136.53,98.12 136.53,98.84 RN24.8
  Bottom 0.203: v137.16,96.53 v137.16,90.18
N$437  (via drill 0.6)
  Top 0.203: IC6.3 111.76,87.64 113.67,89.55 118.75,89.55 121.28,92.09 121.28,93.36 122.56,94.63 135.25,94.63 135.89,95.26 v135.89,96.53 | v135.89,90.18 IC2.6
  Top 0.229: v135.89,96.53 135.89,97.8 135.57,98.12 135.57,98.82 RN24.7
  Bottom 0.203: v135.89,96.53 v135.89,90.18
N$438  (via drill 0.6)
  Top 0.203: IC6.2 110.49,87.64 112.78,89.93 117.86,89.93 120.65,92.72 120.65,93.99 121.92,95.26 133.99,95.26 134.62,95.9 v134.62,96.53 | v134.62,90.18 IC2.7
  Top 0.229: v134.62,96.53 134.62,97.8 134.94,98.12 134.94,98.82 RN24.6
  Bottom 0.203: v134.62,96.53 v134.62,90.18
N$439  (via drill 0.6)
  Top 0.203: IC6.1 109.22,87.64 111.89,90.31 116.59,90.31 120.02,93.74 120.02,94.63 121.28,95.9 132.72,95.9 v133.35,96.53 | v133.35,90.18 IC2.8
  Top 0.229: v133.35,96.53 133.35,97.48 133.99,98.12 133.99,98.84 RN24.5
  Bottom 0.203: v133.35,96.53 v133.35,90.18
N$440
  Top 0.406: RN2.7 79.14,89.78 78.11,90.82 59.58,90.82 R30.C
N$441
  Top 0.406: RN5.1 209.62,91.38 208.91,92.09 182.76,92.09 R16.C
N$442
  Top 0.406: RN8.7 RN7.2
N$443
  Top 0.406: RN7.3 RN8.6
N$444
  Top 0.406: RN8.5 RN7.4
N$445
  Top 0.406: RN5.2 209.15,90.58 208.28,91.45 185.94,91.45 R15.C
N$446
  Top 0.406: RN4.3 77.87,85.97 75.56,88.28 72.28,88.28 R26.C
N$447
  Top 0.406: RN5.4 208.21,88.98 207.01,90.18 192.29,90.18 R13.C
N$448
  Top 0.406: RN5.5 RN6.4
N$449
  Top 0.406: RN7.1 RN8.8
N$450
  Top 0.406: RN8.1 208.35,87.57 206.38,89.55 195.47,89.55 R12.C
N$451
  Top 0.406: RN5.6 RN6.3
N$452
  Top 0.406: RN8.2 207.88,86.77 205.74,88.91 198.64,88.91 R11.C
N$453
  Top 0.406: RN6.2 RN5.7
N$454
  Top 0.406: RN5.8 RN6.1
N$455
  Top 0.406: RN3.4 RN4.5
N$456
  Top 0.406: RN2.5 80.08,91.38 79.38,92.09 53.23,92.09 R32.C
N$458
  Top 0.406: RN5.3 208.68,89.78 207.65,90.82 189.12,90.82 R14.C
N$459
  Top 0.406: RN8.3 207.41,85.97 205.1,88.28 201.81,88.28 R10.C
N$460
  Top 0.406: RN2.8 78.67,88.98 77.47,90.18 62.75,90.18 R29.C
N$461
  Top 0.406: RN4.1 78.81,87.57 76.83,89.55 65.92,89.55 R28.C
N$462
  Top 0.406: RN4.2 78.34,86.77 76.2,88.91 69.1,88.91 R27.C
N$463
  Top 0.406: RN12.4 RN11.5
N$464
  Top 0.305: R25.C 75.05,87.01
  Top 0.406: RN4.4 77.4,85.17 75.56,87.01 75.05,87.01
N$465
  Top 0.406: RN2.1 RN1.8
N$466
  Top 0.406: RN2.2 RN1.7
N$467
  Top 0.406: RN2.3 RN1.6
N$468
  Top 0.406: RN2.4 RN1.5
N$469
  Top 0.406: RN2.6 79.61,90.58 78.74,91.45 56.4,91.45 R31.C
N$470
  Top 0.406: RN8.4 206.94,85.17 205.1,87.01 204.59,87.01 R9.C
N$473
  Top 0.406: RN12.5 206.94,82.49 205.1,80.66 204.59,80.66 R1.C
N$474
  Top 0.406: RN11.6 RN12.3
N$475
  Top 0.406: RN12.6 207.41,81.69 205.1,79.39 201.81,79.39 R2.C
N$476
  Top 0.406: RN12.7 207.88,80.89 205.74,78.75 198.64,78.75 R3.C
N$477
  Top 0.406: RN9.4 RN10.5
N$478
  Top 0.406: RN10.6 RN9.3
N$479
  Top 0.406: RN9.2 RN10.7
N$480
  Top 0.406: RN10.8 RN9.1
N$481
  Top 0.406: RN12.2 RN11.7
N$482
  Top 0.406: RN10.1 208.21,78.68 207.01,77.48 192.29,77.48 R5.C
N$483
  Top 0.406: RN12.8 208.35,80.09 206.38,78.12 195.47,78.12 R4.C
N$484
  Top 0.406: RN10.3 209.15,77.08 208.28,76.21 185.94,76.21 R7.C
N$485
  Top 0.406: RN10.4 209.62,76.28 208.91,75.58 182.76,75.58 R8.C
N$486
  Top 0.406: RN10.2 208.68,77.88 207.65,76.85 189.12,76.85 R6.C
N$487
  Top 0.406: RN14.3 78.97,80.89 76.83,78.75 69.1,78.75 R19.C
N$488
  Top 0.406: RN14.2 78.5,81.69 76.2,79.39 72.28,79.39 R18.C
N$489
  Top 0.406: RN14.1 78.03,82.49 76.2,80.66 75.05,80.66 R17.C
N$490
  Top 0.406: RN16.4 80.72,76.28 80.01,75.58 53.23,75.58 R24.C
N$491
  Top 0.406: RN15.3 RN16.6
N$492
  Top 0.406: RN15.2 RN16.7
N$493
  Top 0.406: RN15.1 88.19,78.68 88.27,78.75 83.42,78.75 RN16.8
N$494
  Top 0.406: RN14.4 79.44,80.09 77.47,78.12 65.92,78.12 R20.C
N$495
  Top 0.406: RN16.3 80.25,77.08 79.38,76.21 56.4,76.21 R23.C
N$496
  Top 0.406: RN16.2 79.78,77.88 78.74,76.85 59.58,76.85 R22.C
N$497
  Top 0.406: RN16.1 79.31,78.68 78.11,77.48 62.75,77.48 R21.C
N$498  (via drill 0.6)
  Top 0.305: IC2.17 v128.27,81.29 | v244.47,81.29 244.47,82.56 245.11,83.2 v247.65,83.2 248.28,83.2 248.92,82.56 IC1.17 | U$13.B1 287.02,93.99 287.02,88.91 287.09,88.98 RN17.5 289.81,88.98 290.51,88.28 v290.51,83.2
  Bottom 0.305: v128.27,81.29 130.18,83.2 136.53,83.2 137.16,83.83 216.85,83.83 217.81,83.2 243.84,83.2 244.47,82.56 v244.47,81.29 | v247.65,83.2 v290.51,83.2
N$500
  Top 0.406: RN11.8 RN12.1
N$501
  Top 0.406: RN13.4 RN14.5
N$502
  Top 0.406: RN14.6 RN13.3
N$503
  Top 0.406: RN13.2 RN14.7
N$504
  Top 0.406: RN14.8 RN13.1
N$505
  Top 0.406: RN4.6 RN3.3
N$506
  Top 0.406: RN4.7 RN3.2
N$507
  Top 0.406: RN4.8 RN3.1
N$514
  Top 0.406: RN15.4 RN16.5
N$525  (via drill 0.5)
  Top 0.229: IC3.7 231.78,74.63 232.41,73.99 260.67,73.99 261.62,74.94 v261.62,77.74 IC1.27 | v266.7,72.09 270.43,72.09 RN18.7
  Bottom 0.229: v266.7,72.09 261.94,72.09 261.62,72.4 v261.62,77.74
N$526
  Top 0.229: IC1.28 262.89,73.99 | 262.89,73.99 262.25,73.35 231.14,73.35 230.5,73.99 IC3.8 | 262.89,73.99 262.89,71.77 263.52,71.13 270.91,71.13 RN18.8
OC_R1_A  (via drill 0.6)
  Top 0.406: IC3.18 v239.4,69.93 239.4,66.69 241.94,64.15 294.64,64.15 295.91,62.88 295.91,46.37 297.81,44.46 328.3,44.46 330.2,42.56 330.2,13.47 K1.2 | RN11.4 227.26,82.49 v227.46,82.31
  Bottom 0.406: v227.46,82.31 239.01,82.31 239.4,81.93 v239.4,69.93
OC_R1_B
  Top 0.203: RN7.5 226.13,85.17 232.73,91.77 237.17,91.77 238.12,92.72 IC4.11
  Top 0.406: IC4.11 238.12,100.34 238.76,100.98 249.56,100.98 250.19,101.61 293.74,101.61 294.64,102.51 294.64,117.86 295.54,118.76 326.39,118.76 327.66,117.49 327.66,112.53 K9.2
OC_R1_C  (via drill 0.6)
  Top 0.406: RN13.8 106.61,82.49 v106.68,82.56 | IC5.18 v119.38,69.86 119.38,67.32 120.65,66.05 160.66,66.05 161.93,64.78 161.93,45.1 158.88,42.05 K17.2
  Bottom 0.406: v106.68,82.56 118.11,82.56 119.38,81.29 v119.38,69.86
OC_R1_D
  Top 0.203: RN3.5 105.48,85.17 111.12,90.82 115.57,90.82 118.11,93.36 IC6.11
  Top 0.406: IC6.11 118.11,100.98 118.75,101.61 161.29,101.61 161.93,102.25 161.93,140.6 K25.2
OC_R2_A  (via drill 0.6)
  Top 0.406: RN11.3 225.66,81.69 v226.06,81.29 | IC3.17 v238.12,69.93 238.17,66.72 241.39,63.51 294,63.51 295.27,62.24 295.27,45.1 296.55,43.83 325.75,43.83 327.53,42.05 K2.2
  Bottom 0.406: v226.06,81.29 236.85,81.29 238.12,80.02 v238.12,69.93
OC_R2_B
  Top 0.203: IC4.12 236.85,93.36 235.9,92.4 232.73,92.4 226.29,85.97 RN7.6
  Top 0.406: IC4.12 236.85,100.98 237.49,101.61 248.92,101.61 249.56,102.25 293.37,102.25 294,102.88 294,118.49 294.9,119.39 325.12,119.39 325.75,120.03 325.75,141.74 K10.2
OC_R2_C  (via drill 0.6)
  Top 0.406: RN13.7 105.01,81.69 v105.41,81.29 | IC5.17 v118.11,69.86 118.11,66.05 119.38,64.78 154.94,64.78 156.21,63.51 156.21,22.87 156.21,22.24 156.21,13.35 158.5,11.06 K18.2
  Bottom 0.406: v105.41,81.29 115.57,81.29 118.11,78.75 v118.11,69.86
OC_R2_D
  Top 0.203: RN3.6 105.01,85.97 110.49,91.45 114.3,91.45 116.84,93.99 IC6.12
  Top 0.406: IC6.12 116.84,101.93 117.47,102.57 158.12,102.57 158.75,103.2 158.75,112.53 K26.2
OC_R3_A  (via drill 0.6)
  Top 0.406: RN11.2 223.92,80.89 v224.79,80.02 | IC3.16 v236.85,69.93 236.85,66.69 240.66,62.88 293.37,62.88 294.64,61.61 294.64,13.98 291.85,11.19 K3.2
  Bottom 0.406: v224.79,80.02 235.59,80.02 236.85,78.75 v236.85,69.93
OC_R3_B
  Top 0.203: RN7.7 226.46,86.77 232.73,93.04 235.27,93.04 235.59,93.36 IC4.13
  Top 0.406: IC4.13 235.59,101.61 236.22,102.25 248.28,102.25 248.92,102.88 290.83,102.88 291.46,103.52 291.46,112.28 K11.2
OC_R3_C  (via drill 0.6)
  Top 0.406: RN13.6 103.27,80.89 v104.14,80.02 | IC5.16 v116.84,69.86 116.84,64.78 118.11,63.51 123.83,63.51 125.73,61.61 125.73,44.84 K19.2
  Bottom 0.406: v104.14,80.02 114.3,80.02 116.84,77.48 v116.84,69.86
OC_R3_D
  Top 0.203: RN3.7 104.54,86.77 109.73,91.96 112.9,91.96 115.57,94.63 IC6.13
  Top 0.406: IC6.13 115.57,102.25 116.84,103.52 125.09,103.52 125.73,104.15 125.73,140.86 K27.2
OC_R4_A  (via drill 0.6)
  Top 0.406: RN11.1 222.18,80.09 v223.52,78.75 | IC3.15 v235.59,69.93 235.59,66.05 239.4,62.24 288.29,62.24 289.56,60.97 289.56,44.46 291.85,42.18 K4.2
  Bottom 0.406: v223.52,78.75 234.31,78.75 235.59,77.48 v235.59,69.93
OC_R4_B
  Top 0.203: RN7.8 226.62,87.57 232.73,93.68 234,93.68 234.31,93.99 IC4.14
  Top 0.406: IC4.14 234.31,102.25 234.95,102.88 247.65,102.88 248.35,103.58 288.93,103.58 289.81,104.47 289.81,141.74 K12.2
OC_R4_C  (via drill 0.6)
  Top 0.406: RN13.5 101.53,80.09 v102.87,78.75 | IC5.15 v115.57,69.86 115.57,63.51 120.02,59.07 120.02,13.86 K20.2
  Bottom 0.406: v102.87,78.75 113.03,78.75 115.57,76.21 v115.57,69.86
OC_R4_D
  Top 0.203: IC6.14 114.3,94.25 112.52,92.47 109.47,92.47 104.65,87.64 89.77,87.64 RN3.8
  Top 0.406: IC6.14 114.3,102.88 116.2,104.79 121.92,104.79 123.19,106.06 123.19,112.41 K28.2
OC_R5_A  (via drill 0.6)
  Top 0.406: RN9.8 221.05,78.68 222.25,77.48 v227.33,77.48 | IC3.14 v234.31,69.93 234.31,65.74 246.38,53.67 246.38,14.11 K5.2
  Bottom 0.406: v227.33,77.48 233.04,77.48 234.31,76.21 v234.31,69.93
OC_R5_B
  Top 0.203: IC4.15 233.04,94.63 232.73,94.31 232.41,94.31 227.08,88.98 RN6.5
  Top 0.406: IC4.15 233.04,102.88 233.68,103.52 241.94,103.52 243.46,105.04 243.46,112.53 K13.2
OC_R5_C  (via drill 0.6)
  Top 0.406: IC5.14 v114.3,69.86 114.3,66.05 113.67,65.42 77.47,65.42 76.83,64.78 76.83,44.59 K21.2 | RN15.8 101.03,78.68 102.23,77.48 v106.68,77.48
  Bottom 0.406: v106.68,77.48 112.39,77.48 114.3,75.58 v114.3,69.86
OC_R5_D
  Top 0.203: IC6.15 113.03,94.12 112.01,93.1 109.09,93.1 105.03,89.04 89.76,89.04 RN1.1
  Top 0.406: IC6.15 113.03,100.34 110.49,102.88 79.38,102.88 77.72,104.53 77.72,140.35 K29.2
OC_R6_A  (via drill 0.6)
  Top 0.406: RN9.7 220.58,77.88 222.25,76.21 v226.06,76.21 | IC3.13 v233.04,69.93 233.04,65.42 241.3,57.16 241.3,44.08 K6.2
  Bottom 0.406: v226.06,76.21 231.78,76.21 233.04,74.94 v233.04,69.93
OC_R6_B
  Top 0.203: RN6.6 226.93,89.78 231.78,94.63 IC4.16
  Top 0.406: IC4.16 231.78,103.52 233.04,104.79 239.4,104.79 241.3,106.69 241.3,141.74 K14.2
OC_R6_C  (via drill 0.6)
  Top 0.406: IC5.13 v113.03,69.86 113.03,67.32 112.39,66.69 72.39,66.69 71.12,65.42 71.12,14.62 74.3,11.44 K22.2 | RN15.7 100.56,77.88 102.23,76.21 v105.41,76.21
  Bottom 0.406: v105.41,76.21 111.76,76.21 113.03,74.94 v113.03,69.86
OC_R6_D
  Top 0.203: IC6.16 111.76,94.12 111.25,93.61 108.71,93.61 105.03,89.93 89.85,89.93 RN1.2
  Top 0.406: IC6.16 111.76,99.71 109.86,101.61 76.2,101.61 74.55,103.26 74.55,112.53 K30.2
OC_R7_A  (via drill 0.6)
  Top 0.406: RN9.6 220.11,77.08 222.25,74.94 v224.79,74.94 | IC3.12 v231.78,69.93 231.78,67.32 231.14,66.69 211.46,66.69 210.19,65.42 210.19,13.35 207.9,11.06 K7.2
  Bottom 0.406: v224.79,74.94 230.5,74.94 231.78,73.67 v231.78,69.93
OC_R7_B
  Top 0.203: RN6.7 226.78,90.58 230.5,94.31 IC4.17
  Top 0.406: IC4.17 230.5,101.61 229.87,102.25 207.65,102.25 207.26,102.63 207.26,112.53 K15.2
OC_R7_C  (via drill 0.6)
  Top 0.406: v111.76,69.86 IC5.12 111.76,68.72 110.87,67.84 41.66,67.83 41.27,67.45 41.27,44.97 K23.2 | RN15.6 100.09,77.08 102.23,74.94 v104.14,74.94
  Bottom 0.406: v104.14,74.94 110.49,74.94 111.76,73.67 v111.76,69.86
OC_R7_D
  Top 0.203: IC6.17 110.49,94.5 110.11,94.12 108.58,94.12 105.03,90.56 89.72,90.56 RN1.3
  Top 0.406: IC6.17 110.49,99.07 109.22,100.34 43.18,100.34 41.53,101.99 41.53,140.6 K31.2
OC_R8_A  (via drill 0.6)
  Top 0.406: RN9.5 219.64,76.28 222.25,73.67 v223.52,73.67 | IC3.11 v230.5,69.93 230.5,68.59 229.87,67.96 205.74,67.96 204.47,66.69 204.47,45.1 K8.2
  Bottom 0.406: v223.52,73.67 229.24,73.67 230.5,72.4 v230.5,69.93
OC_R8_B
  Top 0.203: RN6.8 226.62,91.38 229.24,93.99 IC4.18
  Top 0.406: IC4.18 229.24,100.98 228.6,101.61 206.06,101.61 205.36,102.31 205.36,141.62 K16.2
OC_R8_C  (via drill 0.6)
  Top 0.406: v110.49,69.86 IC5.11 110.49,73.04 109.86,73.67 107.95,73.67 107.31,73.04 107.31,69.86 106.68,69.23 36.2,69.23 35.56,68.59 35.56,13.98 38.35,11.19 K24.2 | RN15.5 99.62,76.28 102.23,73.67 v102.87,73.67
  Bottom 0.406: v102.87,73.67 109.22,73.67 110.49,72.4 v110.49,69.86
OC_R8_D
  Top 0.203: RN1.4 104.96,91.38 107.57,93.99 107.57,94.32 108.97,95.72 IC6.18
  Top 0.406: IC6.18 109.22,97.8 107.95,99.07 40.01,99.07 38.35,100.72 38.35,112.53 K32.2
REG_5V  (via drill 0.5, 0.6, 0.9)
  Top 0.254: 285.75,98.44 285.75,98.12 U$13.A2 | 339.13,37.99 337.95,37.99 v337.19,38.75 | RN26.6 RN26.5 317.12,92.32 317.12,92.85 316.74,93.23 v316.74,93.61
  Top 0.305: IC2.15 v125.73,85.1 126.36,85.1 129.54,81.93 129.54,78.75 | 250.19,85.1 251.46,86.37 252.09,86.37 252.73,87.01 | IC2.9 132.08,87.64 v130.81,86.37 | IC1.18 v250.19,84.47 | IC1.9 252.73,87.01 | 252.73,87.01 253.37,86.37 263.84,86.37 264.16,86.37 265.43,87.64 270.51,87.64 | 270.51,87.64 281.31,87.64 284.48,90.82 285.75,90.82 285.99,90.58 | 286.22,94.79 U$13.B2 U$13.A2 | C1.1 270.6,87.56 270.51,87.64 | 339.13,37.99 RNB1.6
  Top 0.406: C2.1 C3.1 | C4.1 C1.1 | IC2.18 129.54,81.93 130.18,82.56 144.55,82.56 | C8.1 144.55,82.56 | 144.55,82.56 C5.1 144.55,77.08 144.78,76.85 149.54,76.85 149.86,77.16 149.86,77.48 | C6.1 C7.1 265.2,85.33 264.16,86.37 | 149.86,78.75 149.86,78.84 | 149.86,78.84 C3.1 | C3.1 149.86,79.07 149.86,78.84
  Top 0.61: v316.74,93.61 318.52,93.61 321.94,90.18 X10.2
  Top 0.813: H1.1 311.63,67.8 v311.15,67.32 | IC7.4 302.39,69.99 | 302.39,69.99 v302.26,69.86 | 302.39,69.99 299.32,69.99 C10.1
  Top 1.016: 154.94,76.85 150.18,76.85 149.86,77.16 | 149.86,77.48 149.86,78.75 | C24.+ 156.21,78.12 154.94,76.85 | C28.+ 156.21,75.58 154.94,76.85 | C1.1 270.6,79.3 271.4,78.5 275.46,78.5 276.03,77.93 | 276.03,77.93 276.23,77.74 C25.+ | C26.+ 283.85,77.48 283.21,78.12 276.23,78.12 276.03,77.93 | C27.+ 268.61,87.96
  Top 1.27: 285.75,98.12 U$13.B2 285.75,91.13 284.16,91.13 280.99,87.96 268.61,87.96 265.43,87.96 263.84,86.37 253.05,86.37 252.73,86.69 251.78,86.69 250.19,85.1 v250.19,84.47 | H1.1 320.14,66.53 v320.68,66.94
  Bottom 0.254: 344.17,53.99 342.9,52.72 338.45,52.72 337.19,51.45 v337.19,38.75 337.19,50.18 338.45,51.45 342.9,51.45 344.17,52.72 344.17,74.31 344.81,74.94 344.81,89.55 344.17,90.18 v339.47,90.18
  Bottom 0.305: v250.19,84.47 219.07,84.47 218.44,85.1 135.89,85.1 135.25,84.47 133.99,84.47 133.35,85.1 v125.73,85.1 125.73,85.74 126.36,86.37 v130.81,86.37
  Bottom 0.61: FOR_NANO.5V 314.96,95.39 | 314.96,95.39 v316.74,93.61 | 314.96,95.39 314.96,95.26 314.32,94.63 302.89,94.63 301.62,93.36
  Bottom 0.813: v311.15,67.32 302.26,67.32 v302.26,69.86 300.99,71.13 300.99,81.93 302.26,83.2 302.26,92.72 301.62,93.36 v300.36,93.36
  Bottom 1.016: v300.36,93.36 286.38,93.36 285.75,93.99 U$13.B2 | v339.47,90.18 X10.2
REG_12V  (via drill 0.5)
  Top 0.813: BRA2.+ 327.02,71.13 325.12,68.59 317.5,68.59 313.69,72.4 311.4,72.4 v307.21,72.53 IC7.7 | C9.1 299.21,82.44 300.36,81.29 301.62,81.29 302.26,80.66 v302.26,75.58
  Bottom 0.813: v302.26,75.58 302.26,73.67 303.4,72.53 v307.21,72.53
UNREG_12V
  Top 2.54: 331.42,66.05 BRA2.~@1 BRA2.~@2 | 331.42,66.05 U$2.TIP | 331.42,66.05 331.42,61.78 332.36,60.85 341.38,60.85 342.14,60.34 341.94,60.34 X17.2

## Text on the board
tNames: Bank 4 | Bank 2 | 8 | 6 | 4 | 2 | 8 | 6 | 4 | 2 | 7 | 5 | 3 | 1 | 7 | 5 | 3 | 1 | MCP23017 | ANSR32x0 | REV.A | Address: | A1 | A2 | GND | 2016 ControlEverything.com | +5V | SC | SDA | SCL | Address A0=0 | Address A0=1 | 12V DC / Power / Supply | 12V DC / Power / Supply | 12V DC / Power / Supply | 8 | 6 | 4 | 2 | 8 | 6 | 4 | 2 | 7 | 5 | 3 | 1 | 7 | 5 | 3 | 1 | Bank 3 | Bank 1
